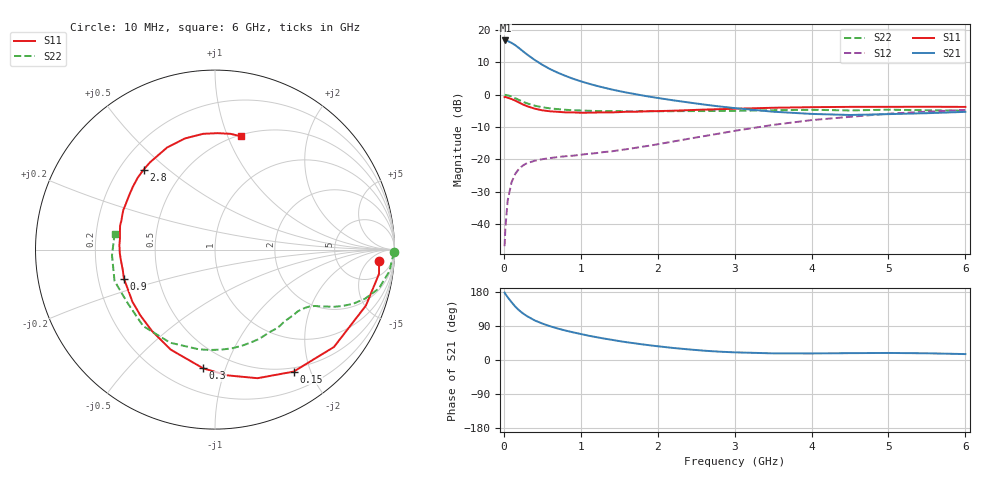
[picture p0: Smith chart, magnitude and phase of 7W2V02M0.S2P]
! Infineon Technologies  Discrete & RF Semiconductors
! BFS17W
! Si NPN RF Bipolar Junction Transistor in SOT323
! VCE = 2 V  IC = 2 mA
! Common Emitter S-Parameters:  August  1999
# GHz  S  MA  R  50
!  f  S11  S21  S12  S22
! GHz  MAG  ANG  MAG  ANG  MAG  ANG  MAG  ANG
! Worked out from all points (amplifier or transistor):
!   36 points, 10 MHz to 6 GHz, reference 50 ohm
!   highest |S21| = 16.7 dB at 20 MHz (marker M1)
!   |S21| within 3 dB of that: start of sweep to 231.4 MHz
!   unconditionally stable (mu >= 1): 800 MHz to end of sweep
!   at 250 MHz: K = 0.36, MSG = 17.6 dB, |S12| = -21.8 dB
!   at 1.4 GHz: K = 1.34, MAG = 6.0 dB, |S12| = -17.5 dB
!   at 6 GHz: K = 1.11, MAG = -2.3 dB, |S12| = -4.7 dB
!   S11 on the Smith chart (normalised r, x): 10 MHz: 14, -11; 150 MHz: 0.44, -1.75; 300 MHz: 0.35, -0.84; 900 MHz: 0.31, -0.14; 2.8 GHz: 0.30, +0.41; 6 GHz: 0.51, +1.11
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0.01  0.9162 -4.0  6.86 177.8  0.0046 87.1  0.9985 -0.9
0.02  0.9238 -8.4  6.862 174.3  0.0088 83.3  0.9897 -2.9
0.05  0.897 -20.3  6.729 165.6  0.0233 79.1  0.9789 -7.1
0.1  0.8566 -39.3  6.295 152.6  0.0444 68.7  0.9388 -13.3
0.15  0.8087 -57.2  5.78 140.6  0.0606 60.3  0.88 -18.1
0.2  0.7547 -71.7  5.209 130.9  0.0723 54.2  0.8254 -21.5
0.25  0.704 -84.4  4.662 122.7  0.0811 48.6  0.7757 -23.9
0.3  0.6648 -95.7  4.19 115.9  0.0877 44.7  0.7369 -25.6
0.4  0.6094 -113.9  3.441 104.6  0.0955 40.2  0.677 -27.9
0.5  0.5736 -127.8  2.894 96.2  0.101 37.8  0.6399 -29.4
0.6  0.554 -138.8  2.484 89.2  0.1052 37.4  0.6146 -31.0
0.7  0.5441 -147.8  2.186 83.1  0.1091 37.3  0.5984 -32.8
0.9  0.5327 -162.3  1.76 73.0  0.1145 38.8  0.575 -36.8
1.1  0.5277 -173.5  1.483 64.2  0.1223 41.5  0.5651 -41.5
1.3  0.5333 177.2  1.286 56.7  0.1302 44.5  0.5568 -46.9
1.6  0.5455 165.8  1.075 46.8  0.1443 49.4  0.5524 -55.2
2.2  0.5658 147.8  0.819 31.8  0.1893 56.9  0.5561 -73.6
2.8  0.5971 131.8  0.659 22.0  0.2513 58.9  0.5601 -93.1
3.5  0.6282 115.2  0.546 17.5  0.3417 55.5  0.5758 -115.7
4.5  0.6484 95.9  0.486 18.1  0.4551 43.9  0.571 -149.1
5.5  0.6508 82.4  0.518 17.7  0.5467 31.9  0.5748 -176.8
6  0.6477 77.3  0.543 15.6  0.5823 26.1  0.5663 171.0
